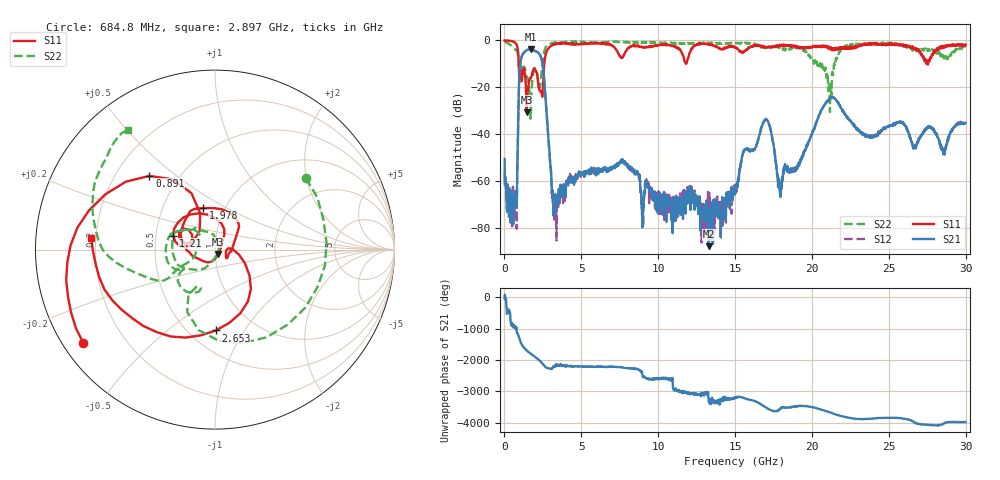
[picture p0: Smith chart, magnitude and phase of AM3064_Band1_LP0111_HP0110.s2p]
# Hz S DB R 50.0
!freq dBS11 angS11 dBS21 angS21 dBS12 angS12 dBS22 angS22
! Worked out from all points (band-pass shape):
!   1600 points, 10 MHz to 29.98 GHz, reference 50 ohm
!   highest |S21| = -3.82 dB at 1.697 GHz (marker M1); lowest = -87.8 dB at 13.28 GHz (marker M2)
!   |S21| within 3 dB of the highest: 1.127 GHz to 2.356 GHz (1.229 GHz wide, 70.6 % of centre)
!   lowest |S11| = -30.7 dB at 1.453 GHz (marker M3), VSWR 1.06, Z = 51.7 - j2.45 ohm
!   |S11| at or under -10 dB: 931.6 MHz to 2.586 GHz (1.655 GHz wide, 94.1 % of centre); 27.52439 GHz to 27.55132 GHz (26.93 MHz wide, 0.0978 % of centre)
!   |S22| runs from -33.4 to -0.3 dB; largest |S21 - S12| = 0.0093
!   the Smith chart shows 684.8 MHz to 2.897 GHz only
!   S11 on the Smith chart (normalised r, x): 684.8 MHz: 0.06, -0.32; 891 MHz: 0.34, +0.40; 1.21 GHz: 0.62, +0.10; 1.978 GHz: 0.79, +0.39; 2.653 GHz: 0.67, -0.76; 2.897 GHz: 0.18, +0.04
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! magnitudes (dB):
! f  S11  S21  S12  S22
! 10 MHz  0.0  -50.6  -56.3  -0.3
! 684.8 MHz  -0.9  -64.3  -69.5  -3.8
! 891 MHz  -5.2  -35.1  -35.0  -6.8
! 1.21 GHz  -12.2  -5.7  -5.7  -11.5
! 1.453 GHz  -30.7  -4.1  -4.1  -15.7
! 1.697 GHz  -15.8  -3.8  -3.9  -33.4
! 1.978 GHz  -12.4  -4.5  -4.5  -12.5
! 2.653 GHz  -6.9  -22.7  -22.8  -3.4
! 2.897 GHz  -3.2  -45.1  -45.3  -1.7
! 3.29 GHz  -1.7  -66.1  -69.7  -0.9
! 5.015 GHz  -1.5  -56.4  -56.5  -0.6
! 7.732 GHz  -6.8  -52.3  -51.5  -0.7
! 10 GHz  -2.1  -70.0  -72.1  -0.9
! 13.28 GHz  -1.9  -87.8  -83.6  -1.4
! 15 GHz  -3.1  -63.1  -64.2  -1.3
! 16.95 GHz  -2.7  -33.9  -33.9  -2.9
! 17.93 GHz  -2.0  -62.1  -65.8  -2.7
! 19.99 GHz  -3.1  -40.0  -39.9  -8.1
! 21.32 GHz  -4.2  -24.2  -24.3  -13.6
! 25 GHz  -1.3  -36.6  -36.8  -1.2
! 28.54 GHz  -2.4  -48.4  -48.6  -6.3
! 29.98 GHz  -1.8  -35.2  -35.3  -2.9
